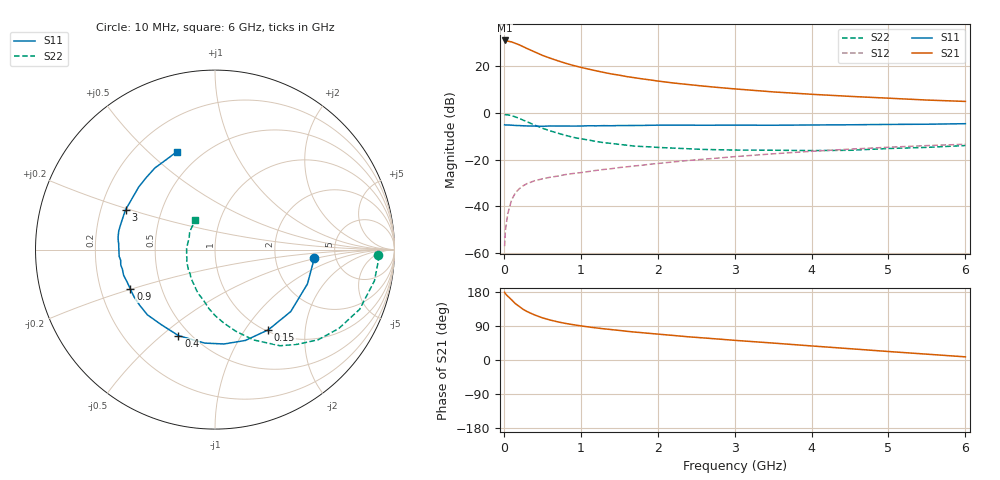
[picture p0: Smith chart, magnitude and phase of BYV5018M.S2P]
! SIEMENS Small Signal Semiconductors
! BFY420
! Si NPN RF SIEGET Grounded Emitter Transistor in MICRO-X
! VCE = 0.5 V  IC = 18 mA
! Common Emitter S-Parameters:  October  1996
# GHz  S  MA  R  50
!  f  S11  S21  S12  S22
! GHz  MAG  ANG  MAG  ANG  MAG  ANG  MAG  ANG
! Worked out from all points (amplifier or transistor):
!   36 points, 10 MHz to 6 GHz, reference 50 ohm
!   highest |S21| = 31.0 dB at 10 MHz (marker M1)
!   |S21| within 3 dB of that: start of sweep to 272.9 MHz
!   unconditionally stable (mu >= 1): start of sweep to 11.17 MHz; 1.604 GHz to end of sweep
!   at 250 MHz: K = 0.31, MSG = 29.8 dB, |S12| = -31.2 dB
!   at 1.4 GHz: K = 0.96, MSG = 20.3 dB, |S12| = -23.9 dB
!   at 6 GHz: K = 1.13, MAG = 7.0 dB, |S12| = -13.4 dB
!   S11 on the Smith chart (normalised r, x): 10 MHz: 3.42, -0.44; 150 MHz: 1.03, -1.29; 400 MHz: 0.43, -0.57; 900 MHz: 0.33, -0.20; 3 GHz: 0.31, +0.19; 6 GHz: 0.37, +0.62
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0.01  0.5541 -4.6  35.42 178.6  0.0014 97.3  0.91 -1.9
0.02  0.5504 -8.5  35.41 175.0  0.003 87.1  0.9119 -4.1
0.05  0.5494 -20.4  34.22 168.6  0.0068 83.2  0.9052 -11.1
0.1  0.5452 -39.3  33 159.0  0.0136 74.3  0.872 -22.4
0.15  0.5367 -56.4  30.7 148.7  0.0194 67.2  0.8179 -32.5
0.2  0.5337 -71.5  28.55 141.3  0.0237 63.2  0.7631 -41.2
0.25  0.5282 -84.5  26.12 133.8  0.0274 58.1  0.6984 -49.1
0.3  0.5241 -96.2  23.89 128.0  0.0305 55.2  0.647 -55.9
0.4  0.5208 -113.0  20.16 118.9  0.0352 50.8  0.5472 -66.9
0.5  0.5144 -125.8  17.04 111.4  0.0386 48.7  0.4695 -75.7
0.6  0.5233 -136.0  14.84 105.6  0.0418 47.4  0.4125 -83.1
0.7  0.5218 -143.4  13.04 100.7  0.0442 46.9  0.3678 -89.9
0.9  0.5205 -154.8  10.36 93.2  0.0503 47.0  0.2995 -100.8
1.1  0.5288 -164.3  8.64 87.2  0.0554 47.7  0.2618 -110.9
1.3  0.532 -170.7  7.325 82.3  0.0614 47.7  0.2298 -119.7
1.6  0.5351 -178.9  5.96 75.7  0.07 47.8  0.2029 -131.9
2.2  0.5462 169.0  4.363 64.8  0.0889 46.5  0.1758 -151.0
3  0.5453 156.0  3.255 51.9  0.1154 42.6  0.1598 -171.2
3.5  0.5427 148.2  2.808 44.7  0.1327 39.5  0.1583 177.5
4.5  0.5549 133.6  2.252 29.8  0.1671 30.3  0.1579 155.7
5.5  0.5706 118.1  1.878 15.4  0.1989 20.1  0.1823 133.6
6  0.5857 111.2  1.755 8.3  0.2129 14.9  0.1995 124.8
